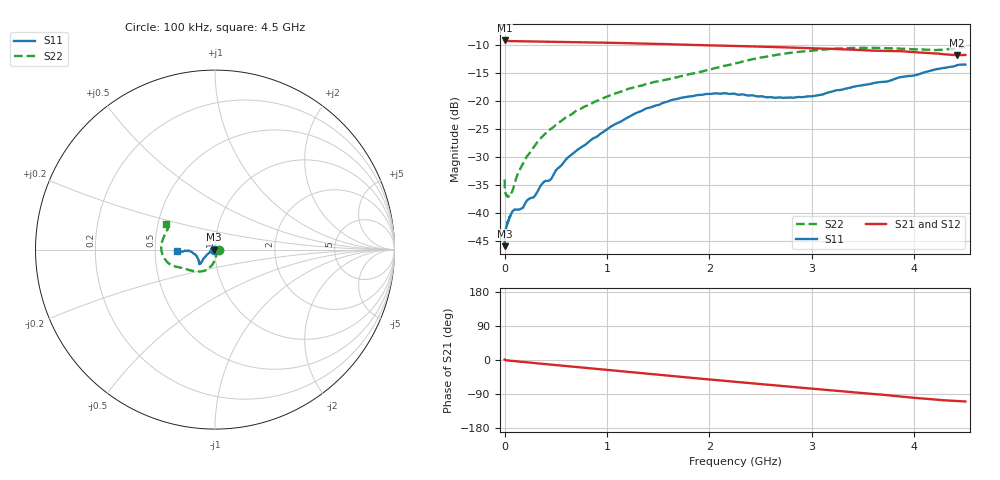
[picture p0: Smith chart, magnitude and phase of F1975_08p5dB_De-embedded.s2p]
! Integrated Device Technology
! Corporate Headquarters
! 6024 Silver Creek Valley Road
! San Jose, CA 95138  USA
! Phone:  1-408-284-8200
! Toll Free:  1-800-223-1366
! Webpage:  http://www.idt.com/
! Timing and RF Division
! 515 Groton Road, Suite 102
! Westford, MA 01886-6024
! Device:  F1975
! Description: 6-bit, 75 ohm, 0.5 dB Digital Step Attenuator
! Frequency:  5.0 MHz -  3.00 GHz
! Package:  4x4 mm QFN Plastic Package: 20 pin
! Ports:  2 RF, 11 DC
!  Pin  1  = D5 (16 dB)
!  Pin  2  = RF1  =  Port 1
!  Pin  3  = Serial Data In (DATA)
!  Pin  4  = Serial Clock (CLK)
!  Pin  5  = Serial Latch Enable (LE)
!  Pin  6  = VDD
!  Pin  7  = NC
!  Pin  8  = NC
!  Pin  9  = NC
!  Pin 10  = GND
!  Pin 11  = GND
!  Pin 12  = NC
!  Pin 13  = VMODE
!  Pin 14  = RF2  =  Port 2
!  Pin 15  = D4 (8 dB)
!  Pin 16  = D3 (4 dB)
!  Pin 17  = D2 (2 dB)
!  Pin 18  = NC
!  Pin 19  = D1 (1 dB)
!  Pin 20  = D0 (0.5 dB)
! State:  17
! Atten State:  8.5 dB
! Voltage:  +3.30 Volts
! Current:  0.565 mA
! Data:  The device was measured on a F1975 evaluation board which has
!  individual transmission lines to the RF pins.  Data was collected
!  using a calibrated network analyzer.  The evaluation board was
!  de-embedded using Automatic Fixture Removal (AFR).
!  The reference plane is the edge of the package pin.
! Misc:
!  Action Tracker AT0415
! Date Measured:  2018-02-08
! Date:  2018-03-26  MJV
! Note:
!  Integrated Device Technology supplies this data as a sample of measured
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# GHz S dB R 75
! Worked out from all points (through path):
!   291 points, 100 kHz to 4.5 GHz, reference 75 ohm
!   highest |S21| = -9.14 dB at 100 kHz (marker M1); lowest = -11.8 dB at 4.42 GHz (marker M2)
!   group delay of S21, straight-line fit = 68.9 ps
!   lowest |S11| = -46.0 dB at 100 kHz (marker M3), VSWR 1.01, Z = 74.2 - j0.0103 ohm
!   |S11| at or under -10 dB: start of sweep to end of sweep
!   |S22| runs from -37.1 to -10.2 dB; largest |S21 - S12| = 0.00016
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0.0001  -45.96 -179.2  -9.14 1.2  -9.14 1.2  -34.05 -0.5
0.0008  -44.41 -174.3  -9.18 1.0  -9.18 1.0  -35.18 -4.2
0.004  -43.60 -173.9  -9.20 0.5  -9.20 0.5  -35.95 -6.8
0.017  -42.58 -171.7  -9.23 -0.7  -9.23 -0.7  -36.88 -19.8
0.055  -40.59 -168.0  -9.26 -1.8  -9.26 -1.8  -36.90 -43.0
0.08  -39.66 -162.5  -9.27 -2.5  -9.27 -2.5  -35.88 -57.4
0.14  -39.41 -155.7  -9.30 -4.1  -9.30 -4.1  -32.54 -69.8
0.22  -37.75 -158.8  -9.32 -6.2  -9.32 -6.2  -29.82 -77.4
0.32  -36.24 -159.9  -9.35 -8.8  -9.35 -8.8  -27.32 -84.8
0.38  -34.52 -155.9  -9.37 -10.4  -9.37 -10.4  -26.14 -86.8
0.44  -34.19 -155.0  -9.38 -11.9  -9.38 -11.9  -25.11 -88.4
0.6  -30.43 -155.5  -9.43 -16.1  -9.43 -16.0  -22.88 -95.4
0.76  -28.12 -150.3  -9.48 -20.2  -9.47 -20.2  -21.21 -100.8
1.06  -24.32 -145.3  -9.57 -28.0  -9.57 -27.9  -18.75 -110.2
1.52  -20.57 -138.2  -9.76 -39.6  -9.76 -39.6  -16.41 -126.1
1.88  -18.93 -136.2  -9.96 -48.5  -9.96 -48.5  -14.85 -140.3
2.26  -18.75 -139.2  -10.13 -57.6  -10.13 -57.6  -13.21 -152.5
2.64  -19.40 -149.9  -10.32 -66.9  -10.32 -66.9  -11.78 -160.8
3.02  -19.08 -164.7  -10.55 -76.0  -10.54 -76.0  -10.93 -169.3
3.76  -16.36 -177.2  -11.00 -93.3  -11.00 -93.3  -10.54 170.3
4.42  -13.57 -176.5  -11.77 -108.2  -11.77 -108.2  -10.45 153.9
4.5  -13.46 -178.5  -11.74 -109.5  -11.73 -109.5  -10.19 152.6
